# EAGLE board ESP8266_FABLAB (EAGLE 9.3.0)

Size 100 x 80 mm. Coordinates in mm from the lower left corner, seen from the top.
Outline: 0,0 100,0 100,80 0,80 0,0
Copper layers (1*16): Top 0.035mm / dielectric 1.5mm / Bottom 0.035mm
Design rules "default": minimum track width 6mil, minimum drill 0.35mm, track to track 6mil, track to pad 6mil, pad to pad 6mil, via to via 6mil, smd to smd 6mil, copper to edge 40mil, drill to drill 6mil, minimum pad ring 10mil, minimum via ring 8mil, stop-mask expansion 4mil, vias tented up to drill 0mil, thermal gap 10mil

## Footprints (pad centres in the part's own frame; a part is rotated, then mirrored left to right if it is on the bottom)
C1206 = smd 1.6 x 1.8: 1 -1.4,0; 2 1.4,0
SOT223 = smd 1.499 x 2.007: 1 -2.261,-3.15; 2 0.025,-3.15; 3 2.311,-3.15 | smd 3.81 x 2.007: 4 0,3.15
R1206 = smd 1.6 x 1.803: 1 -1.422,0; 2 1.422,0
6MM_SWITCH = smd 2.286 x 1.524: 1 -3.302,2.286; 2 3.302,2.286; 3 -3.302,-2.286; 4 3.302,-2.286
XCVR_ESP8266-12E/ESP-12E = smd 2 x 1.2: 1 -7.5,7; 2 -7.5,5; 3 -7.5,3; 4 -7.5,1; 5 -7.5,-1; 6 -7.5,-3; 7 -7.5,-5; 8 -7.5,-7; 15 7.5,-7; 16 7.5,-5; 17 7.5,-3; 18 7.5,-1; 19 7.5,1; 20 7.5,3; 21 7.5,5; 22 7.5,7 | smd 1.1 x 1.7: 9 -5,-8.5; 10 -3,-8.5; 11 -1,-8.5; 12 1,-8.5; 13 3,-8.5; 14 5,-8.5
1X06SMD = smd 2.54 x 1.27: 1 0,6.35; 2 0,3.81; 3 0,1.27; 4 0,-1.27; 5 0,-3.81; 6 0,-6.35
LED1206 = smd 1.6 x 1.803: 1 -1.422,0; 2 1.422,0

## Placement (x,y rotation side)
C1  [C1206]  22.86,31.75 0 top
C2  [C1206]  19.05,17.78 90 top
IC2  REG1117  [SOT223]  38.1,22.86 270 top
R1  [R1206]  19.05,24.13 180 top
S1  [6MM_SWITCH]  19.05,44.45 180 top
U1  ESP8266-12E/ESP-12E  [XCVR_ESP8266-12E/ESP-12E]  36.83,41.91 0 top
U$1  FTDI-SMD-HEADER  [1X06SMD]  36.83,11.43 90 top
U$2  LED  [LED1206]  16.51,35.56 90 top

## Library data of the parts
C1 = fab; C1: 0.1uf
C2 = fab; C2: 0.1uf
IC2 = burr-brown; MPN: REG1117; OC_FARNELL: 1097566; OC_NEWARK: 14P6981
R1 S1 U$1 U$2 = fab
U1 = ESP8266-12E_ESP-12E; AVAILABILITY: Unavailable; DESCRIPTION: This WiFi module has a 32-bit MCU micro and clock speeds supporting 80 MHz or 160 MHz. Supports the RTOS and integrated Wi-Fi MAC/BB/RF/PA/LNA, and has an on-board antenna.; MF: AI-Thinker; MP: ESP8266-12E/ESP-12E; PACKAGE: None; PRICE: None

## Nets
3.3V: C2.1 IC2.2 U1.1 U1.3 U1.8
5V: C1.1 IC2.3 U$1.3
GND: C1.2 C2.2 IC2.1 S1.1 S1.2 U1.15 U1.16 U$1.1 U$2.2
LED: R1.1 U1.13
MODE: S1.3 S1.4 U1.18
N$1: R1.2 U$2.1
RXD: U1.22 U$1.5
TXD: U1.21 U$1.4

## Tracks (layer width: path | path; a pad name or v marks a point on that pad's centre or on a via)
3.3V  (4 unrouted)
5V  (2 unrouted)
GND  (8 unrouted)
LED  (1 unrouted)
MODE  (2 unrouted)
N$1  (1 unrouted)
RXD  (1 unrouted)
TXD  (1 unrouted)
